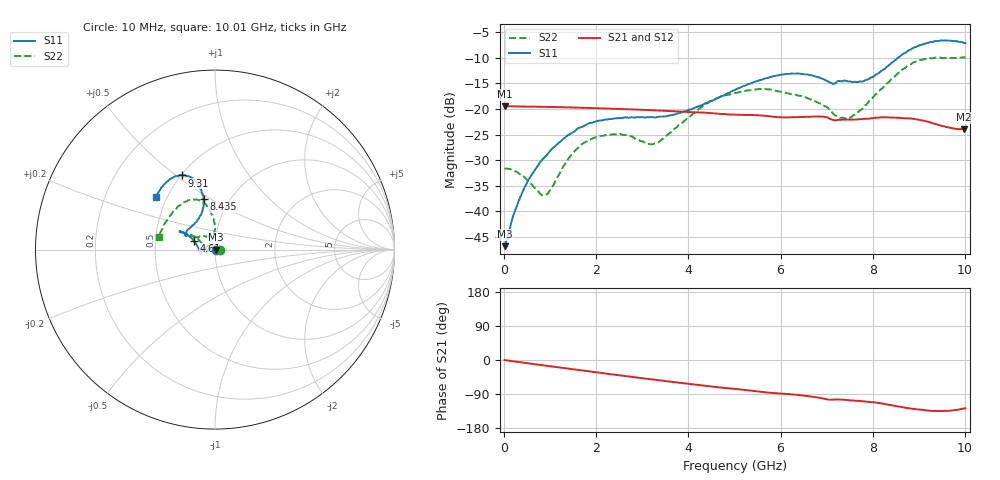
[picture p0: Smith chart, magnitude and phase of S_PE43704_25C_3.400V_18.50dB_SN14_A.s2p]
! Device ID: PE43704
! Dir: z:\PE43704\PE43704_Char_1_20130516\PE43704\AMB\3p400V\18p50dB
! Serial: 14
! Insertion: A
! Impedance: 50 ohm
! Temp: Amb
! VDD: 3.400V
! Attenuation Step: 18.50dB
! IDD: 1.140390e-01mA
#  Hz  S  RI  R  50
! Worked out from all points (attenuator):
!   401 points, 10 MHz to 10.01 GHz, reference 50 ohm
!   highest |S21| = -19.46 dB at 10 MHz (marker M1); lowest = -23.9 dB at 9.985 GHz (marker M2)
!   lowest |S11| = -46.8 dB at 10 MHz (marker M3), VSWR 1.01, Z = 50.5 + j0.036 ohm
!   |S11| at or under -10 dB: start of sweep to 8.547 GHz
!   |S22| runs from -36.8 to -9.9 dB; largest |S21 - S12| = 0.0013
!   S11 on the Smith chart (normalised r, x): 10 MHz: 1.01, +0.00; 4.61 GHz: 0.79, +0.08; 8.435 GHz: 0.76, +0.46; 9.31 GHz: 0.51, +0.53; 10.01 GHz: 0.44, +0.32
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1e7  0.00457 0.000357  0.1064 -0.000313  0.1064 -0.000327  0.0261 0.000237
2.35e8  0.00255 0.00979  0.1056 -0.00745  0.1056 -0.00746  0.0236 0.00707
4.35e8  -0.00248 0.0167  0.1045 -0.0134  0.1047 -0.0135  0.0182 0.012
8.85e8  -0.0243 0.0239  0.1013 -0.0266  0.1013 -0.0265  -0.00332 0.0143
1.41e9  -0.0542 0.0148  0.0951 -0.0407  0.0952 -0.0407  -0.0334 0.000593
1.685e9  -0.0665 0.00555  0.091 -0.0476  0.0912 -0.0475  -0.0441 -0.0101
2.36e9  -0.0788 -0.0153  0.0791 -0.0622  0.0792 -0.0621  -0.0508 -0.025
3.135e9  -0.0812 -0.0181  0.0626 -0.0748  0.0625 -0.0749  -0.045 -0.00818
3.36e9  -0.0832 -0.0121  0.0573 -0.0776  0.0574 -0.0775  -0.0475 0.0019
4.61e9  -0.117 0.0479  0.0285 -0.0855  0.0287 -0.0856  -0.1059 0.0697
5.01e9  -0.1368 0.0691  0.0207 -0.0854  0.021 -0.0854  -0.1223 0.0735
5.685e9  -0.1752 0.0952  0.00655 -0.0851  0.00676 -0.0852  -0.1323 0.0828
6.685e9  -0.1898 0.0952  -0.00994 -0.0834  -0.00989 -0.0835  -0.1011 0.069
7.135e9  -0.157 0.0795  -0.0197 -0.0756  -0.0199 -0.0759  -0.0539 0.073
7.46e9  -0.1464 0.1147  -0.0217 -0.0759  -0.0216 -0.0758  -0.0215 0.0802
7.835e9  -0.0984 0.1631  -0.0267 -0.0758  -0.0264 -0.0757  -0.00135 0.1088
8.36e9  -0.063 0.2614  -0.0395 -0.0728  -0.0393 -0.073  -0.0125 0.1852
8.435e9  -0.064 0.2806  -0.0413 -0.0715  -0.0414 -0.0715  -0.0209 0.1991
8.86e9  -0.1031 0.3759  -0.0501 -0.0625  -0.0492 -0.0629  -0.0754 0.2704
9.31e9  -0.1833 0.4134  -0.0507 -0.0515  -0.0509 -0.0517  -0.1648 0.2663
9.985e9  -0.3226 0.2995  -0.0391 -0.0501  -0.04 -0.0499  -0.3079 0.0791
1.001e10  -0.3279 0.2918  -0.0386 -0.0507  -0.0399 -0.0509  -0.3119 0.0693
